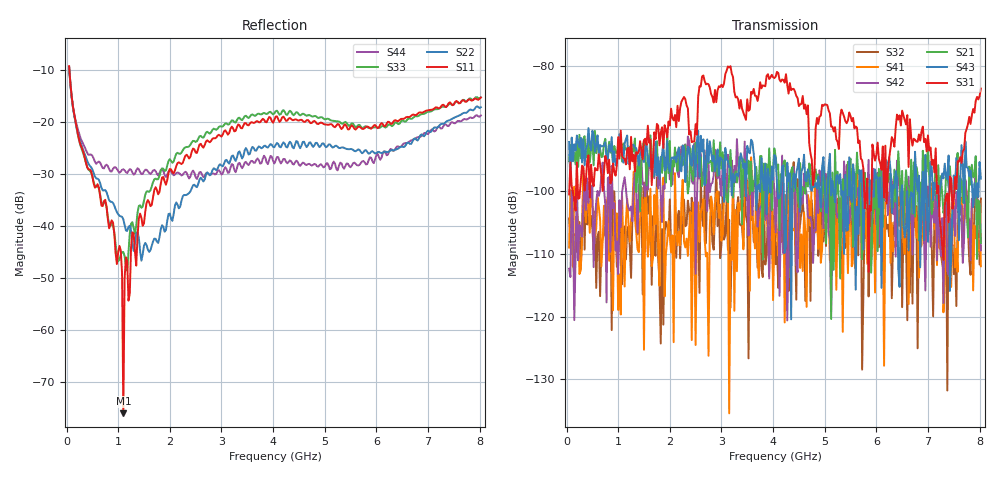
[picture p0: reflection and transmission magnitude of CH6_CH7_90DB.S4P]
!Agilent Technologies,E5071C,MY46316741,A.11.02
!Date: Mon Jun 01 10:19:19 2026
!Data & Calibration Information:
!1:CH6 INPUT 2:CH6 OUTPUT 3:CH7 INPUT 4:CH7 OUTPUT
!Freq	S11:SOLT4(ON)	S12:SOLT4(ON)	S13:SOLT4(ON)	S14:SOLT4(ON)
!	S21:SOLT4(ON)	S22:SOLT4(ON)	S23:SOLT4(ON)	S24:SOLT4(ON)
!	S31:SOLT4(ON)	S32:SOLT4(ON)	S33:SOLT4(ON)	S34:SOLT4(ON)
!	S41:SOLT4(ON)	S42:SOLT4(ON)	S43:SOLT4(ON)	S44:SOLT4(ON)
!PortZ  Port1:50+j0  Port2:50+j0  Port3:50+j0  Port4:50+j0
!Above PortZ is port z conversion or system Z0 setting when saving the data.
!When reading, reference impedance value at option line is always used.
# Hz S dB R 50
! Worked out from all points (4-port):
!   320 points, 50 MHz to 8.025 GHz, reference 50 ohm
!   strongest paths, dB at 50 MHz, 2.05 GHz, 4.05 GHz, 6.05 GHz, 8.025 GHz:
!     S31: -100.5, -88.3, -81.7, -94.8, -83.6
!     S43: -92.1, -94.6, -94.6, -102.5, -98.0
!     S21: -95.2, -95.1, -94.4, -96.4, -108.2
!     S42: -112.3, -98.9, -106.5, -108.3, -109.4
!     S41: -109.0, -107.0, -102.2, -103.3, -111.9
!     S32: -104.3, -107.3, -111.6, -108.9, -101.1
!   lowest |S11| = -75.9 dB at 1.1 GHz (marker M1), VSWR 1.00, Z = 50 + j0.0124 ohm
!   |S11| at or under -10 dB: 55.17 MHz to end of sweep
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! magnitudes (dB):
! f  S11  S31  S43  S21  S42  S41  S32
! 50 MHz  -9.3  -100.5  -92.1  -95.2  -112.3  -109.0  -104.3
! 1.05 GHz  -44.6  -90.3  -93.2  -92.8  -105.7  -119.6  -111.3
! 1.075 GHz  -49.0  -94.3  -93.2  -95.2  -100.1  -100.6  -114.8
! 1.1 GHz  -75.9  -94.7  -95.4  -92.4  -98.8  -108.6  -110.7
! 1.15 GHz  -46.0  -95.7  -91.7  -93.4  -99.6  -104.7  -110.8
! 2 GHz  -29.0  -89.5  -96.9  -92.0  -98.1  -107.3  -101.3
! 8.025 GHz  -15.3  -83.6  -98.0  -108.2  -109.4  -111.9  -101.1
